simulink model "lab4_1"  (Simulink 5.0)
settings: Solver=FixedStepDiscrete  StartTime=0.0  StopTime=25*T  FixedStep=T  RelTol=1e-3
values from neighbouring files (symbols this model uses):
  Fsamp = 10e3    (= 10000)    [lab4_4.m]
  T = 1/Fsamp    (= 0.0001)    [lab4_4.m]

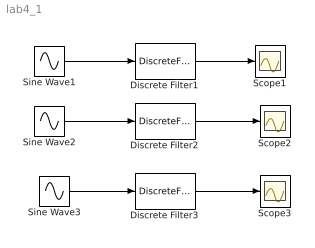
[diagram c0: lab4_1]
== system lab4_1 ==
  Discrete Filter1 : DiscreteFilter  Denominator=[1 0.5]  SampleTime=1/Fsamp
  Discrete Filter2 : DiscreteFilter  Denominator=[1 0.5]  SampleTime=1/Fsamp
  Discrete Filter3 : DiscreteFilter  Denominator=[1 0.5]  SampleTime=1/Fsamp
  Scope1 : Scope
  Scope2 : Scope
  Scope3 : Scope
  Sine Wave1 : Sin  Frequency=2*pi*2e3  SampleTime=T
  Sine Wave2 : Sin  Frequency=2*pi*12e3  SampleTime=T
  Sine Wave3 : Sin  Frequency=2*pi*8e3  SampleTime=T
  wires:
  Sine Wave1/1 -> Discrete Filter1/1
  Discrete Filter1/1 -> Scope1/1
  Sine Wave2/1 -> Discrete Filter2/1
  Discrete Filter2/1 -> Scope2/1
  Sine Wave3/1 -> Discrete Filter3/1
  Discrete Filter3/1 -> Scope3/1
